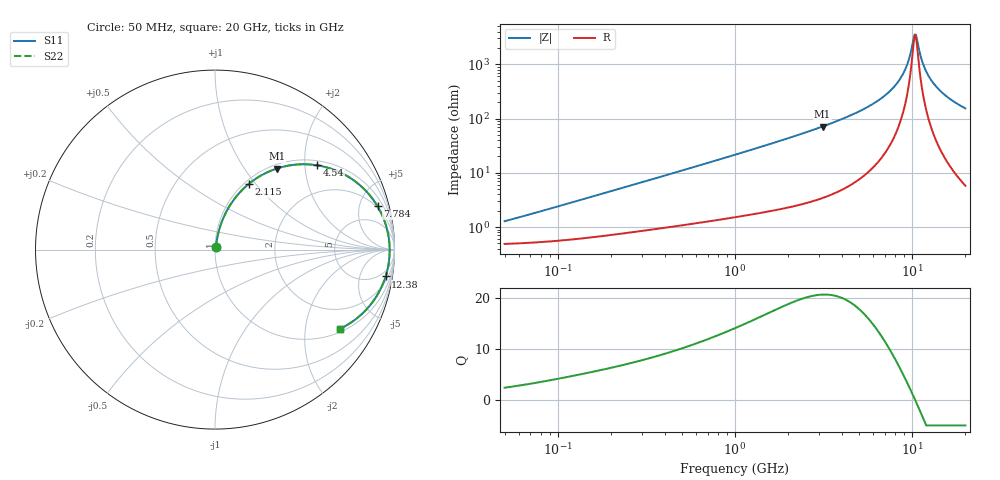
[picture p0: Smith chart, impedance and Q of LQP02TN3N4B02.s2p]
!Murata Part Number: LQP02TN3N4B02
!These Parameters are Measured in Series Mode Connection
!  o--[Z]--o
!Port1  Port2
!  o-------o
!Freq. Start=50[MHz] Stop=20[GHz], 401[Steps]
# Hz S RI R 50
!Freq.(Hz) S11(Real) S11(Imag) S21(Real) S21(Imag) S12(Real) S12(Imag) S22(Real) S22(Imag)
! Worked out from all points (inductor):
!   401 points, 50 MHz to 20 GHz, reference 50 ohm
!   read as one part in series: L = 3.74 nH near 64.5 MHz
!   highest Q = 20.7 at 3.122 GHz (marker M1), where L = 3.63 nH
!   self-resonance near 10.35 GHz
!   S11 on the Smith chart (normalised r, x): 50 MHz: 1.01, +0.02; 2.115 GHz: 1.05, +0.92; 4.54 GHz: 1.12, +2.32; 7.784 GHz: 1.81, +7.20; 12.38 GHz: 3, -12; 20 GHz: 1.12, -3.07
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5e7  0.00501 0.0118  0.995 -0.0118  0.995 -0.0118  0.00501 0.0118
1.364002e8  0.00711 0.0311  0.9929 -0.0311  0.9929 -0.0311  0.00711 0.0311
3.721004e8  0.0158 0.0801  0.9842 -0.0801  0.9842 -0.0801  0.0158 0.0801
1e9  0.057 0.1992  0.943 -0.1992  0.943 -0.1992  0.057 0.1992
2.114743e9  0.1875 0.3652  0.8125 -0.3652  0.8125 -0.3652  0.1875 0.3652
2.728004e9  0.2804 0.4255  0.7196 -0.4255  0.7196 -0.4255  0.2804 0.4255
3.121702e9  0.3439 0.4515  0.6561 -0.4515  0.6561 -0.4515  0.3439 0.4515
4.539627e9  0.5702 0.4695  0.4298 -0.4695  0.4298 -0.4695  0.5702 0.4695
6.034176e9  0.764 0.3922  0.236 -0.3922  0.236 -0.3922  0.764 0.3922
7.442007e9  0.8853 0.2728  0.1147 -0.2728  0.1147 -0.2728  0.8853 0.2728
7.784049e9  0.906 0.2409  0.094 -0.2409  0.094 -0.2409  0.906 0.2409
8.516016e9  0.9398 0.1718  0.0602 -0.1718  0.0602 -0.1718  0.9398 0.1718
9.178299e9  0.9595 0.1098  0.0405 -0.1098  0.0405 -0.1098  0.9595 0.1098
9.600142e9  0.9672 0.0713  0.0328 -0.0713  0.0328 -0.0713  0.9672 0.0713
1.019291e10  0.9726 0.019  0.0274 -0.019  0.0274 -0.019  0.9726 0.019
1.034674e10  0.9731 0.00581  0.0269 -0.00581  0.0269 -0.00581  0.9731 0.00581
1.066139e10  0.9729 -0.0205  0.0271 0.0205  0.0271 0.0205  0.9729 -0.0205
1.149051e10  0.9663 -0.086  0.0337 0.086  0.0337 0.086  0.9663 -0.086
1.238412e10  0.9508 -0.1497  0.0492 0.1497  0.0492 0.1497  0.9508 -0.1497
1.354865e10  0.9214 -0.222  0.0786 0.222  0.0786 0.222  0.9214 -0.222
1.504638e10  0.8738 -0.2978  0.1262 0.2978  0.1262 0.2978  0.8738 -0.2978
2e10  0.6959 -0.4416  0.3041 0.4416  0.3041 0.4416  0.6959 -0.4416
